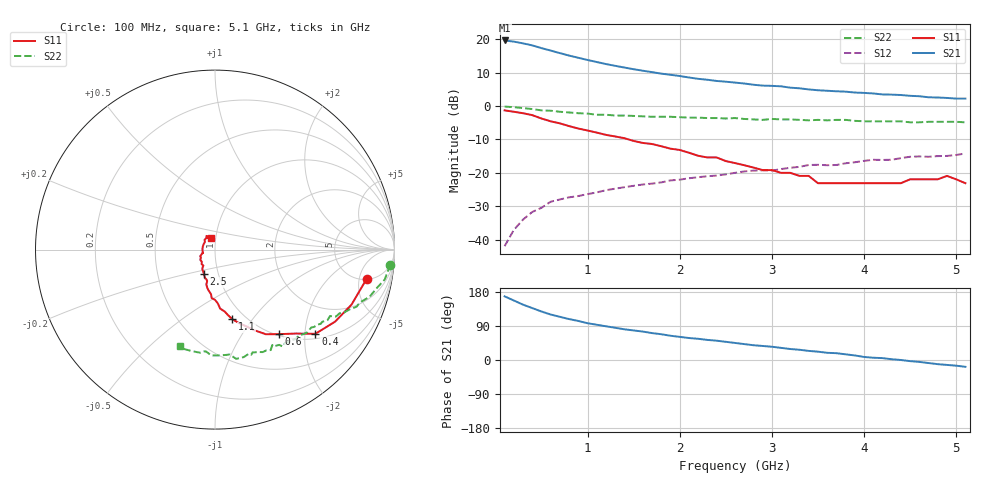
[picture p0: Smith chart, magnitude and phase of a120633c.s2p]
!  INA-12063 S PARAMETERS
!  Vd = 3 V  Id = 4.5 mA  LAST UPDATED 10-07-96
# ghz s ma r 50
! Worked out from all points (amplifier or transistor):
!   51 points, 100 MHz to 5.1 GHz, reference 50 ohm
!   highest |S21| = 19.6 dB at 100 MHz (marker M1)
!   |S21| within 3 dB of that: start of sweep to 596.8 MHz
!   unconditionally stable (mu >= 1): 1.066 GHz to end of sweep
!   at 900 MHz: K = 0.88, MSG = 20.7 dB, |S12| = -26.9 dB
!   at 2.6 GHz: K = 1.37, MAG = 9.9 dB, |S12| = -20.0 dB
!   at 5.1 GHz: K = 1.42, MAG = 4.3 dB, |S12| = -14.2 dB
!   S11 on the Smith chart (normalised r, x): 100 MHz: 5.09, -6.41; 400 MHz: 1.13, -2.26; 600 MHz: 1.02, -1.48; 1.1 GHz: 0.87, -0.80; 2.5 GHz: 0.85, -0.24; 5.1 GHz: 0.95, +0.12
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0.1  0.86 -11.0  9.56 168.0  0.008 79.0  0.98 -5.0
0.2  0.82 -22.0  9.18 157.0  0.014 73.0  0.96 -10.0
0.3  0.78 -31.0  8.65 146.0  0.02 71.0  0.93 -13.0
0.4  0.73 -40.0  8.07 137.0  0.026 68.0  0.9 -17.0
0.5  0.65 -46.0  7.34 128.0  0.03 62.0  0.86 -20.0
0.6  0.59 -53.0  6.75 120.0  0.037 61.0  0.85 -22.0
0.8  0.5 -64.0  5.68 108.0  0.043 56.0  0.8 -26.0
1  0.43 -72.0  4.88 97.0  0.048 52.0  0.77 -29.0
1.1  0.4 -76.0  4.55 93.0  0.051 52.0  0.74 -30.0
1.4  0.33 -85.0  3.76 81.0  0.061 50.0  0.72 -35.0
1.8  0.25 -95.0  3.05 68.0  0.072 48.0  0.69 -41.0
2  0.22 -101.0  2.81 61.0  0.079 45.0  0.68 -44.0
2.5  0.15 -114.0  2.31 48.0  0.095 42.0  0.65 -53.0
2.6  0.14 -118.0  2.24 45.0  0.1 40.0  0.66 -55.0
2.8  0.12 -125.0  2.08 39.0  0.108 36.0  0.63 -59.0
3.1  0.1 -137.0  1.97 32.0  0.114 35.0  0.63 -63.0
3.4  0.09 -156.0  1.77 24.0  0.131 30.0  0.61 -70.0
3.5  0.07 -166.0  1.72 22.0  0.132 26.0  0.62 -71.0
4  0.07 167.0  1.57 8.0  0.151 24.0  0.59 -82.0
4.3  0.07 146.0  1.48 2.0  0.157 20.0  0.59 -89.0
4.9  0.09 122.0  1.32 -13.0  0.179 10.0  0.58 -103.0
5.1  0.07 110.0  1.29 -18.0  0.195 9.0  0.57 -110.0
